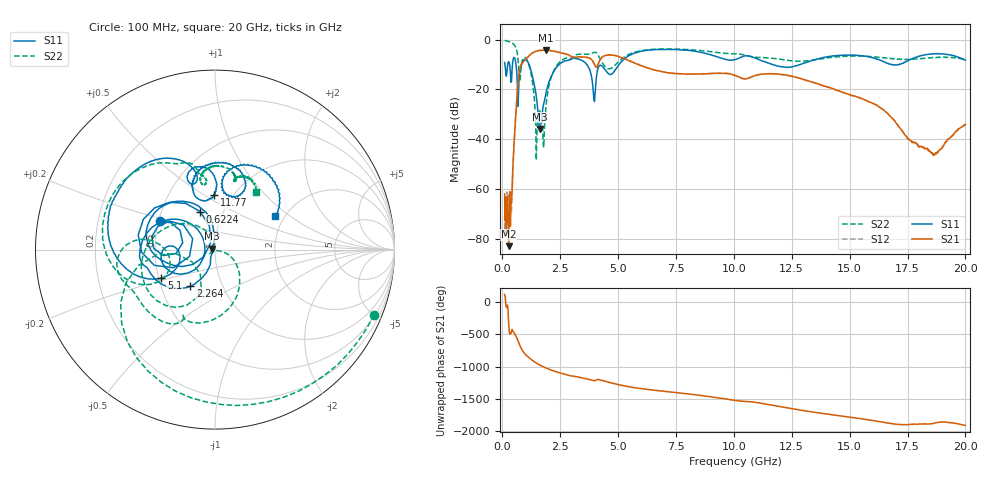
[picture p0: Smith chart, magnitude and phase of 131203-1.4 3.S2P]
!  2-Port S-parameters saved by WinCal
! VAR MeasName=S-Parameters (CALIBRATED_DATA) read from VNA (N5244A)
! VAR MeasDate=4/4/2013 3:56:27 PM
! VAR NAME=131203-1.4 3
! VAR FILENAME=131203-1.4 3.S2P
! VAR DATE=4/4/2013 3:56:27 PM
! VAR PHYS_PORTS=1,2
# Hz S MA R 50
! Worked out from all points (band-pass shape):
!   801 points, 100 MHz to 20 GHz, reference 50 ohm
!   highest |S21| = -4.28 dB at 1.891 GHz (marker M1); lowest = -83.0 dB at 274.1 MHz (marker M2)
!   |S21| within 3 dB of the highest: 1.079 GHz to 3.698 GHz (2.619 GHz wide, 110 % of centre); 4.292 GHz to 5.16 GHz (867.9 MHz wide, 18.4 % of centre)
!   lowest |S11| = -35.9 dB at 1.617 GHz (marker M3), VSWR 1.03, Z = 48.5 + j0.517 ohm
!   |S11| at or under -10 dB: 1.153 GHz to 2.458 GHz (1.305 GHz wide, 72.3 % of centre); 3.645 GHz to 5.047 GHz (1.402 GHz wide, 32.3 % of centre); 11.65 GHz to 12.87 GHz (1.218 GHz wide, 9.94 % of centre)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
!   |S22| runs from -48.4 to -0.4 dB; largest |S21 - S12| = 0.0033
!   S11 on the Smith chart (normalised r, x): 100 MHz: 0.51, +0.18; 622.4 MHz: 0.78, +0.35; 2.264 GHz: 0.70, -0.31; 5.1 GHz: 0.52, -0.18; 11.77 GHz: 0.83, +0.55; 20 GHz: 1.80, +0.78
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1e8  0.3459 153.0  0.0007996 108.3  0.0002036 -132.6  0.957 -22.2
2.74125e8  0.3595 168.4  7.112e-05 42.9  0.0001125 -23.1  0.9158 -59.6
3.73625e8  0.1384 153.9  0.0004794 -132.6  0.0004389 -106.7  0.8778 -81.8
6.22375e8  0.2273 111.2  0.05904 165.0  0.05915 165.1  0.6039 -150.5
8.71125e8  0.3531 -178.3  0.342 -34.6  0.3428 -34.6  0.3875 -123.6
1.119875e9  0.3425 128.2  0.454 -133.8  0.455 -133.8  0.342 166.4
1.44325e9  0.08789 92.4  0.578 139.8  0.5794 139.8  0.01906 95.2
1.617375e9  0.01605 160.6  0.6021 103.2  0.6039 103.2  0.03692 -139.3
1.766625e9  0.04584 -120.9  0.6084 76.8  0.6099 76.7  0.007988 -132.9
1.891e9  0.08539 -107.7  0.6112 57.3  0.613 57.2  0.04694 -16.2
2.264125e9  0.2463 -123.9  0.5801 6.7  0.5815 6.7  0.2562 -58.8
3.43325e9  0.3799 163.1  0.4455 -93.6  0.4466 -93.6  0.5077 -140.1
3.955625e9  0.06421 153.5  0.3355 -136.8  0.3358 -136.9  0.5493 -163.9
4.204375e9  0.3015 -164.9  0.3785 -122.8  0.3802 -123.0  0.4228 172.3
5.099875e9  0.3381 -152.1  0.4433 154.3  0.445 154.1  0.3868 -151.0
6.741625e9  0.6301 155.5  0.2342 67.9  0.2346 67.7  0.6434 164.9
1.005e10  0.3956 110.5  0.1907 -82.6  0.191 -82.9  0.5167 110.8
1.176638e10  0.3032 90.8  0.2046 -162.9  0.2047 -163.1  0.4153 98.8
1.338325e10  0.38 109.9  0.1396 101.3  0.1396 100.9  0.3834 101.9
1.669162e10  0.3249 66.9  0.03075 -72.5  0.03077 -72.4  0.4163 74.0
1.863188e10  0.5179 63.8  0.00499 -74.9  0.005028 -75.2  0.4295 70.5
2e10  0.3846 28.9  0.01985 -107.2  0.01978 -107.5  0.3964 54.5
